(* Logix 5000 AddOnInstructionDefinition export AMCI_3202_AOP_Reset_Errors; software revision 20.03 *)

ADD_ON_INSTRUCTION AMCI_3202_AOP_Reset_Errors   (* revision 1.0, vendor AMCI, ExecuteEnableInFalse *)
VAR_INPUT
   axis_status_bits : INT; {required}
   channel_number : INT; {required}
END_VAR
VAR_OUTPUT
   EN : BOOL; {access Read Only, visible}
END_VAR
VAR_IN_OUT
   AMCI_3202_output_data : AM:1756_3202:O:0; {required}
END_VAR
VAR
   command_data_block : DINT[8]; {access None}
END_VAR

ROUTINE EnableInFalse   (* ladder *)
END_ROUTINE

ROUTINE Logic   (* ladder *)
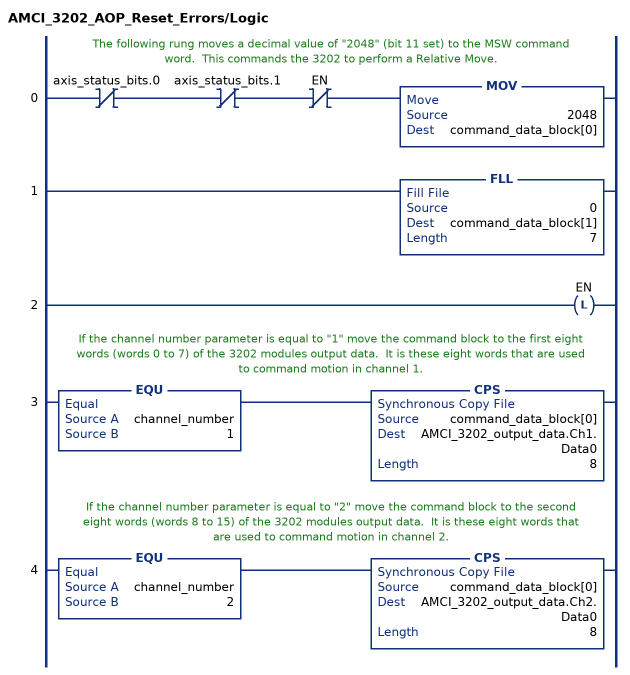
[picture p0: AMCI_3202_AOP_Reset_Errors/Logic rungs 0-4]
   // The following rung moves a decimal value of "2048" (bit 11 set) to the MSW command word.  This commands the 3202 to perform a Relative Move.
   0: XIO(axis_status_bits.0)XIO(axis_status_bits.1)XIO(EN)MOV(2048,command_data_block[0]);
   1: FLL(0,command_data_block[1],7);
   2: OTL(EN);
   // If the channel number parameter is equal to "1" move the command block to the first eight words (words 0 to 7) of the 3202 modules output data.  It is these eight words that are used to command motion in channel 1.
   3: EQU(channel_number,1)CPS(command_data_block[0],AMCI_3202_output_data.Ch1.Data0,8);
   // If the channel number parameter is equal to "2" move the command block to the second eight words (words 8 to 15) of the 3202 modules output data.  It is these eight words that are used to command motion in channel 2.
   4: EQU(channel_number,2)CPS(command_data_block[0],AMCI_3202_output_data.Ch2.Data0,8);
END_ROUTINE
END_ADD_ON_INSTRUCTION
